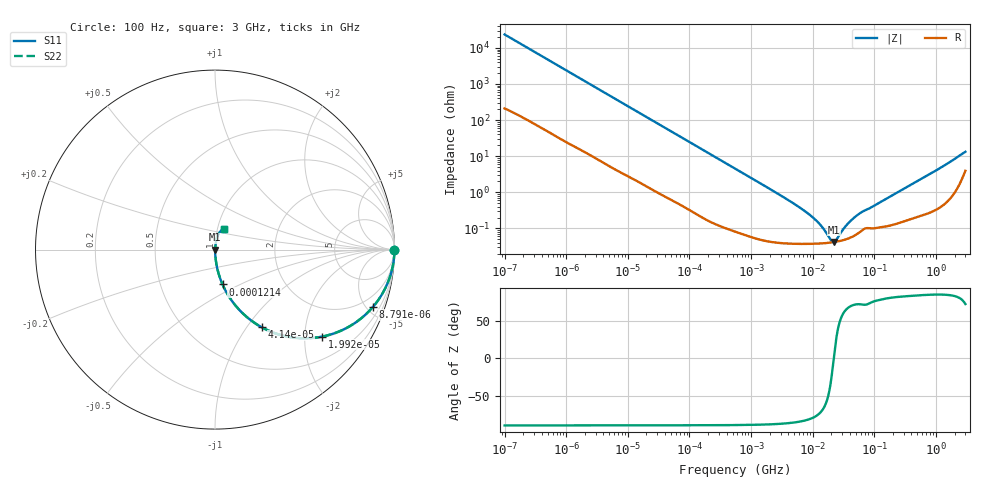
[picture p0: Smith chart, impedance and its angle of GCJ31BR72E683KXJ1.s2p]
!Murata Part Number: GCJ31BR72E683KXJ1
!These Parameters are Measured in Series Mode Connection
!Data Generated on Mar 13, 2026
!  o--ll--o
!Port1  Port2
!  o------o
!Operation Temp=25[degC], DC Bias Voltage=0[V]
!Freq. Start=100[Hz] Stop=3[GHz] 401[Steps]
# Hz S RI R 50
!Freq.(Hz) S11(Real) S11(Imag) S21(Real) S21(Imag) S12(Real) S12(Imag) S22(Real) S22(Imag)
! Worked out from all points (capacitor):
!   401 points, 100 Hz to 3 GHz, reference 50 ohm
!   read as one part in series: C = 67.7 nF near 109 Hz
!   lowest |Z| = 41.9 mohm at 22.19 MHz (marker M1)
!   series resonance near 21.93 MHz, so ESL is about 780 pH
!   S11 on the Smith chart (normalised r, x): 100 Hz: open; 8.791 kHz: 1.06, -5.50; 19.92 kHz: 1.03, -2.44; 41.4 kHz: 1.01, -1.18; 121.4 kHz: 1.01, -0.41; 3 GHz: 1.08, +0.25
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100  0.9999 -0.00426  5.63e-05 0.00426  5.63e-05 0.00426  0.9999 -0.00426
1788  0.9937 -0.0742  0.00634 0.0742  0.00634 0.0742  0.9937 -0.0742
4610  0.9628 -0.1839  0.0372 0.1839  0.0372 0.1839  0.9628 -0.1839
8791  0.8805 -0.3187  0.1195 0.3187  0.1195 0.3187  0.8805 -0.3187
12951  0.7755 -0.4114  0.2245 0.4114  0.2245 0.4114  0.7755 -0.4114
19917  0.5979 -0.4844  0.4021 0.4844  0.4021 0.4844  0.5979 -0.4844
31977  0.3701 -0.4768  0.6299 0.4768  0.6299 0.4768  0.3701 -0.4768
41399  0.2616 -0.4333  0.7384 0.4333  0.7384 0.4333  0.2616 -0.4333
66468  0.1234 -0.3225  0.8766 0.3225  0.8766 0.3225  0.1234 -0.3225
121426  0.042 -0.1943  0.958 0.1943  0.958 0.1943  0.042 -0.1943
547723  0.00288 -0.0453  0.9971 0.0453  0.9971 0.0453  0.00288 -0.0453
4141163  0.000413 -0.00586  0.9996 0.00586  0.9996 0.00586  0.000413 -0.00586
9794414  0.000378 -0.00205  0.9996 0.00205  0.9996 0.00205  0.000378 -0.00205
1.382041e7  0.000385 -0.00109  0.9996 0.00109  0.9996 0.00109  0.000385 -0.00109
1.950129e7  0.000405 -0.000268  0.9996 0.000268  0.9996 0.000268  0.000405 -0.000268
2.21892e7  0.000418 2.75e-05  0.9996 -2.75e-05  0.9996 -2.75e-05  0.000418 2.75e-05
2.418395e7  0.000429 0.000224  0.9996 -0.000224  0.9996 -0.000224  0.000429 0.000224
3.562563e7  0.000508 0.00114  0.9995 -0.00114  0.9995 -0.00114  0.000508 0.00114
5.026954e7  0.00067 0.00207  0.9993 -0.00207  0.9993 -0.00207  0.00067 0.00207
1.751444e8  0.00124 0.0073  0.9988 -0.0073  0.9988 -0.0073  0.00124 0.0073
9.384596e8  0.00447 0.0373  0.9955 -0.0373  0.9955 -0.0373  0.00447 0.0373
3e9  0.0519 0.1153  0.9481 -0.1153  0.9481 -0.1153  0.0519 0.1153
